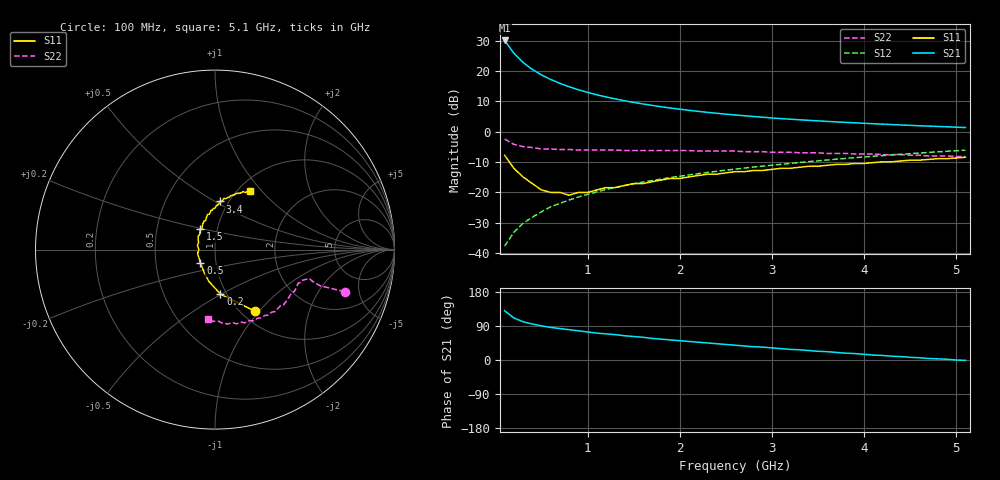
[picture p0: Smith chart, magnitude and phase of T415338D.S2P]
!AT-41533
!S and NOISE PARAMETERS at Vce=8V  Ic=25mA.  LAST UPDATED 01-25-95
# ghz s ma r 50
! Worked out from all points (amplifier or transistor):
!   51 points, 100 MHz to 5.1 GHz, reference 50 ohm
!   highest |S21| = 30.1 dB at 100 MHz (marker M1)
!   |S21| within 3 dB of that: start of sweep to 171.5 MHz
!   unconditionally stable (mu >= 1): 430.3 MHz to 2.073 GHz
!   at 900 MHz: K = 1.05, MAG = 16.3 dB, |S12| = -21.5 dB
!   at 2.6 GHz: K = 0.96, MSG = 8.9 dB, |S12| = -12.3 dB
!   at 5.1 GHz: K = 0.86, MSG = 3.7 dB, |S12| = -6.1 dB
!   lowest NFmin = 1.30 dB at 100 MHz
!   S11 on the Smith chart (normalised r, x): 100 MHz: 1.15, -0.95; 200 MHz: 0.94, -0.50; 500 MHz: 0.84, -0.13; 1.5 GHz: 0.83, +0.19; 3.4 GHz: 0.91, +0.53; 5.1 GHz: 1.14, +0.87
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0.1  0.41 -57.0  32.03 130.0  0.013 73.0  0.76 -18.0
0.2  0.25 -83.0  19.76 111.0  0.022 73.0  0.62 -19.0
0.3  0.18 -101.0  13.92 101.0  0.031 75.0  0.57 -18.0
0.4  0.14 -116.0  10.69 95.0  0.039 75.0  0.55 -17.0
0.5  0.11 -138.0  8.664 90.0  0.048 76.0  0.52 -19.0
0.6  0.1 -156.0  7.29 86.0  0.058 76.0  0.52 -19.0
0.7  0.1 -166.0  6.286 83.0  0.066 76.0  0.51 -20.0
0.8  0.09 179.0  5.522 80.0  0.075 76.0  0.51 -21.0
0.9  0.1 168.0  4.938 77.0  0.084 75.0  0.5 -22.0
1  0.1 156.0  4.46 74.0  0.093 74.0  0.5 -24.0
1.1  0.11 149.0  4.071 71.0  0.102 74.0  0.5 -25.0
1.2  0.12 142.0  3.757 69.0  0.112 73.0  0.5 -26.0
1.4  0.13 130.0  3.248 64.0  0.13 71.0  0.49 -29.0
1.5  0.14 126.0  3.054 62.0  0.139 71.0  0.49 -31.0
1.8  0.16 115.0  2.585 55.0  0.166 68.0  0.49 -34.0
2.2  0.19 104.0  2.172 47.0  0.204 64.0  0.48 -40.0
2.6  0.22 96.0  1.893 39.0  0.242 61.0  0.48 -46.0
2.8  0.23 92.0  1.785 35.0  0.262 58.0  0.47 -50.0
3.4  0.27 84.0  1.544 25.0  0.322 52.0  0.45 -60.0
3.5  0.27 82.0  1.513 23.0  0.332 51.0  0.45 -62.0
4.3  0.32 71.0  1.315 10.0  0.415 42.0  0.42 -78.0
5.1  0.38 59.0  1.174 -1.0  0.497 32.0  0.39 -96.0
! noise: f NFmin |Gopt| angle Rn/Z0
0.1  1.3  0.07  13  0.16
0.9  1.6  0.12  164  0.12
1.8  1.9  0.36  -134  0.15
2.4  2.1  0.51  -109  0.28
